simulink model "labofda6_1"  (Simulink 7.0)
settings: Solver=ode45  StartTime=0.0  StopTime=5.0  RelTol=1e-3

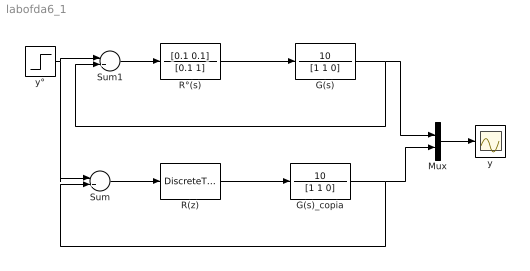
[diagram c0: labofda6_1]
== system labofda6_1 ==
  G(s) : TransferFcn  Numerator=10  Denominator=[1 1 0]
  G(s)_copia : TransferFcn  Numerator=10  Denominator=[1 1 0]
  Mux : Mux  Inputs=2
  R(z) : DiscreteTransferFcn  Numerator=[1.1 -1]  Denominator=[2 -1]  SampleTime=0.1
  R°(s) : TransferFcn  Numerator=[0.1 0.1]  Denominator=[0.1 1]
  Sum : Sum  Inputs=|+-
  Sum1 : Sum  Inputs=|+-
  y : Scope
  y° : Step  Time=0  SampleTime=0
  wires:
  Sum1/1 -> R°(s)/1
  y°/1 -> Sum1/1, Sum/1
  G(s)/1 -> Mux/1, Sum1/2
  Mux/1 -> y/1
  R°(s)/1 -> G(s)/1
  Sum/1 -> R(z)/1
  G(s)_copia/1 -> Sum/2, Mux/2
  R(z)/1 -> G(s)_copia/1
